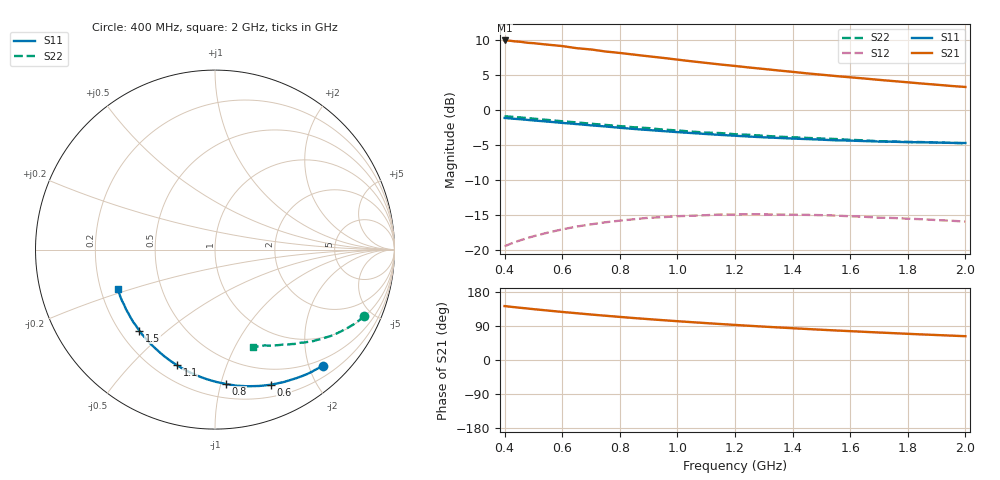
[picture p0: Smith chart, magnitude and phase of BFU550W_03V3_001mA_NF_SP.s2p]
! Filename:  P:\Prog\Test\Noise\ATS_data\Testdata_Net\06 Compressed Noise after Statistics\BFU550W_APM2013_11_D05_03p3V_001mA_NF_CM01_D.sf
! Date/Time: Tue 26/Mar/2013 16:25:21
! BFU550W_APM2013_11_D05_03p3V_1to35mA_NF_CM01_Bias1_R.sf
! Noise Parameter Data File
! BFU550W_APM2013_11_D05_03p3V_1to35mA_NF_CM01
! Date/time: Mon Mar 25 12:16:07 2013
! freq range =  0.4000 to  2.0000 GHz, 37 points
! bias range =  0.9950 to 34.9900 mA, 9 points
! bias supplies used: 1 1 0 0 0 0
! VAR bias_mode= 1  ! Specify V_out, I_out
! VAR bias_var = 1  ! Bias variable = I_out
! VAR V_out= 3.300000
! VAR I_out= 0.995000
! VAR V_in= 0.776300
! VAR I_in= 0.010200
! Device data file deembeded for feedlines and parallel
! Original file: \06 Compressed Noise after Statistics\BFU550W_APM2013_11_D05_03p3V_001mA_NF_CM01_R.sf
! Feed-files: PR019V01_070313_Feed1.s2p, PR019V01_070313_Feed2.s2p
! Parallel-file: PR019V01_070313_Par.s2p
# MHz S MA R 50
!  Freq-MHz  S11-mag  S11-arg  S21-mag  S21-arg  S12-mag  S12-arg  S22-mag  S22-arg
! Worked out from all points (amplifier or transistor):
!   37 points, 400 MHz to 2 GHz, reference 50 ohm
!   highest |S21| = 10.0 dB at 400 MHz (marker M1)
!   |S21| within 3 dB of that: start of sweep to 1.054 GHz
!   unconditionally stable (mu >= 1): nowhere
!   at 500 MHz: K = 0.21, MSG = 13.8 dB, |S12| = -18.0 dB
!   at 1.1 GHz: K = 0.43, MSG = 10.9 dB, |S12| = -15.0 dB
!   at 2 GHz: K = 0.82, MSG = 9.6 dB, |S12| = -15.9 dB
!   lowest NFmin = 0.45 dB at 420 MHz
!   S11 on the Smith chart (normalised r, x): 400 MHz: 0.38, -2.24; 600 MHz: 0.32, -1.44; 800 MHz: 0.30, -1.04; 1.1 GHz: 0.29, -0.68; 1.5 GHz: 0.28, -0.41; 2 GHz: 0.27, -0.18
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400  0.883 -47.0  3.161 142.3  0.1071 60.9  0.9087 -24.0
420  0.8754 -49.2  3.145 140.6  0.1112 59.6  0.9022 -25.0
460  0.8626 -53.5  3.084 137.4  0.119 57.2  0.8886 -26.9
480  0.8554 -55.5  3.041 135.8  0.1226 56.1  0.8813 -27.9
500  0.8479 -57.6  3.023 134.2  0.126 54.9  0.8737 -28.8
600  0.8144 -67.6  2.883 126.8  0.1411 49.7  0.8366 -33.0
650  0.7987 -72.1  2.785 123.4  0.1479 47.4  0.8214 -34.8
700  0.7821 -76.8  2.726 120.0  0.1533 45.0  0.8033 -36.9
750  0.7675 -81.1  2.637 116.8  0.1587 43.0  0.7878 -38.4
800  0.7514 -85.4  2.574 113.7  0.163 40.9  0.7724 -40.2
850  0.7368 -89.6  2.503 110.7  0.1669 39.0  0.7575 -41.7
950  0.7114 -97.4  2.373 105.1  0.1726 35.6  0.7297 -44.8
1050  0.6887 -104.7  2.243 99.8  0.1768 32.6  0.7054 -47.4
1100  0.6782 -108.2  2.185 97.3  0.1783 31.2  0.6944 -48.6
1200  0.6593 -115.0  2.078 92.5  0.1803 28.7  0.6758 -51.2
1250  0.6502 -118.3  2.025 90.2  0.1815 27.5  0.6692 -52.1
1350  0.6358 -124.4  1.93 86.0  0.1802 25.7  0.649 -54.6
1500  0.6179 -133.1  1.8 79.9  0.1784 23.3  0.63 -57.9
1650  0.6035 -141.3  1.69 74.3  0.1737 21.9  0.6109 -61.2
1750  0.597 -146.2  1.62 70.9  0.1703 21.5  0.5997 -63.2
1850  0.5915 -151.0  1.555 67.5  0.1668 21.2  0.5939 -65.3
2000  0.585 -158.0  1.471 62.8  0.1605 22.0  0.5815 -68.5
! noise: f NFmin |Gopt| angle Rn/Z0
400  0.4999  0.6505  31.01  0.2975
460  0.5538  0.6459  36.68  0.3082
600  0.582  0.6684  45.13  0.3165
800  0.6423  0.6409  61.1  0.258
1000  0.7806  0.6317  73.51  0.2834
1200  0.8176  0.6481  87.29  0.2311
1400  0.8047  0.6344  102.6  0.1811
1600  0.6724  0.6141  116.6  0.1285
1800  1.041  0.6668  129.9  0.1021
2000  1.083  0.6344  142.4  0.0864
